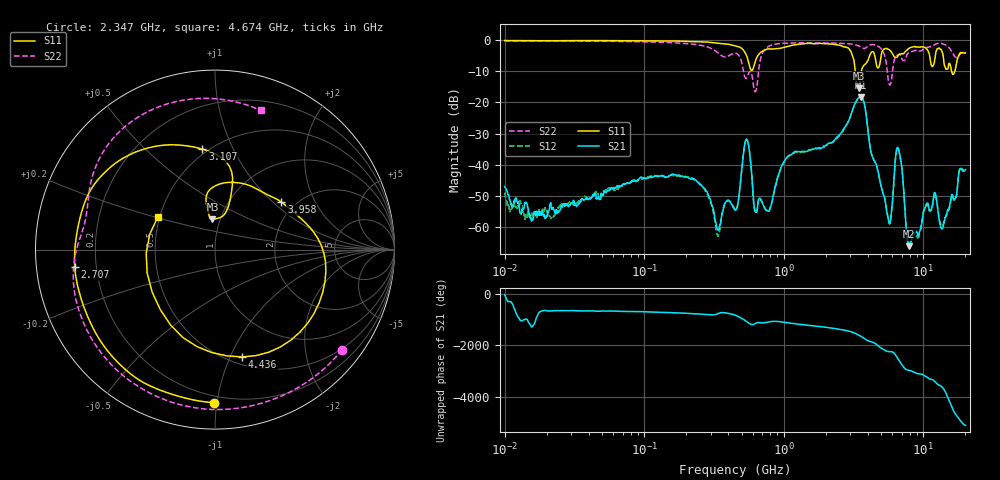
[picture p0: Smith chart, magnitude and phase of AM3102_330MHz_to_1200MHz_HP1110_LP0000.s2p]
! Date/Time: Tue, Sep 11, 2018 5:22 PM
! Network Analyzer: Agilent Technologies E8362B Rev: A.07.50.63
! Sweep from 0.010 to 20.000 GHz, 1601 Points, Sweep Type: LOG
! Power Supply: 4.949 V, 0.001 A
# Hz S DB R 50
!freq MagS11 AngS11 MagS21 AngS21 MagS12 AngS12 MagS22 AngS22
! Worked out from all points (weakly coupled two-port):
!   1601 points, 10 MHz to 20 GHz, reference 50 ohm
!   highest |S21| = -18.26 dB at 3.549 GHz (marker M1); lowest = -66.2 dB at 7.92 GHz (marker M2)
!   lowest |S11| = -15.5 dB at 3.432 GHz (marker M3), VSWR 1.41, Z = 46 + j15.9 ohm
!   |S11| at or under -10 dB: 3.25 GHz to 3.596 GHz (345.7 MHz wide, 10.1 % of centre); 15.92 GHz to 16.8 GHz (886.6 MHz wide, 5.42 % of centre)
!   |S22| runs from -16.5 to -0.2 dB; largest |S21 - S12| = 0.0072
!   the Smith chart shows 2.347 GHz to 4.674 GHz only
!   S11 on the Smith chart (normalised r, x): 2.347 GHz: 0.16, -0.98; 2.707 GHz: 0.12, -0.06; 3.107 GHz: 0.47, +0.77; 3.958 GHz: 1.70, +1.13; 4.436 GHz: 0.57, -1.11; 4.674 GHz: 0.49, +0.21
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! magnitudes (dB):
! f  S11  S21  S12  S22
! 10 MHz  0.0  -47.1  -49.0  -0.2
! 35.55 MHz  -0.1  -51.1  -51.3  -0.2
! 126.4 MHz  -0.2  -43.7  -43.8  -0.6
! 252.9 MHz  -0.5  -46.5  -46.4  -1.6
! 336.3 MHz  -0.9  -60.9  -62.9  -3.9
! 447.2 MHz  -1.8  -54.7  -54.2  -4.2
! 538.2 MHz  -4.7  -31.9  -31.9  -12.2
! 623.6 MHz  -6.9  -54.9  -55.4  -16.5
! 765 MHz  -2.8  -54.9  -55.1  -2.1
! 1.59 GHz  -1.0  -35.1  -35.1  -0.8
! 2.347 GHz  -1.4  -31.7  -32.1  -0.9
! 2.707 GHz  -2.1  -28.2  -28.6  -1.0
! 3.107 GHz  -5.0  -22.3  -22.5  -1.2
! 3.432 GHz  -15.5  -18.5  -18.6  -1.8
! 3.549 GHz  -11.8  -18.3  -18.2  -2.1
! 3.958 GHz  -6.8  -26.9  -26.8  -2.1
! 4.436 GHz  -4.2  -38.7  -38.6  -1.4
! 4.674 GHz  -8.7  -41.1  -41.2  -1.8
! 5.652 GHz  -2.9  -58.4  -58.5  -13.7
! 6.612 GHz  -4.8  -34.8  -34.9  -4.5
! 7.92 GHz  -2.5  -66.2  -65.9  -3.9
! 20 GHz  -4.0  -41.6  -42.1  -3.8
